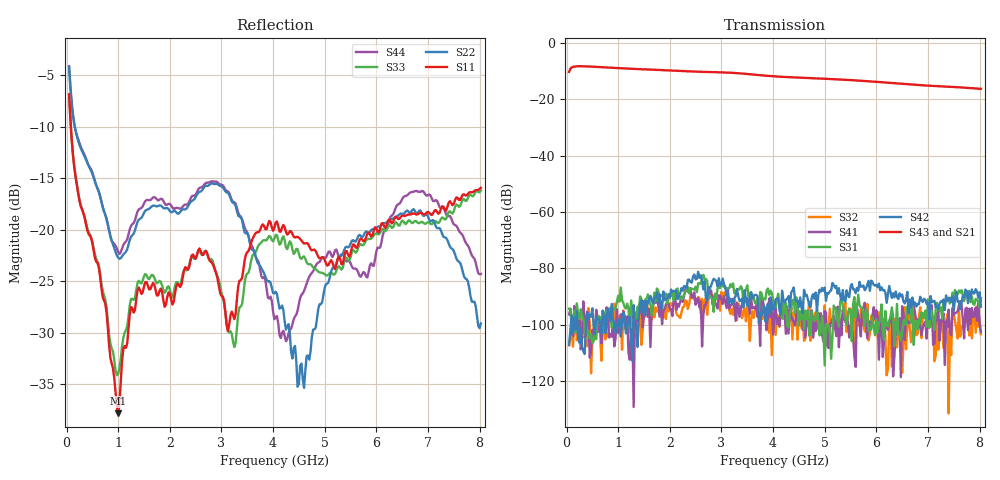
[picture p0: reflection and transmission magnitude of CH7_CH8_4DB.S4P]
!Agilent Technologies,E5071C,MY46316741,A.11.02
!Date: Mon Jun 01 10:29:19 2026
!Data & Calibration Information:
!1:CH7 INPUT 2:CH7 OUTPUT 3:CH8 INPUT 4:CH8 OUTPUT
!Freq	S11:SOLT4(ON)	S12:SOLT4(ON)	S13:SOLT4(ON)	S14:SOLT4(ON)
!	S21:SOLT4(ON)	S22:SOLT4(ON)	S23:SOLT4(ON)	S24:SOLT4(ON)
!	S31:SOLT4(ON)	S32:SOLT4(ON)	S33:SOLT4(ON)	S34:SOLT4(ON)
!	S41:SOLT4(ON)	S42:SOLT4(ON)	S43:SOLT4(ON)	S44:SOLT4(ON)
!PortZ  Port1:50+j0  Port2:50+j0  Port3:50+j0  Port4:50+j0
!Above PortZ is port z conversion or system Z0 setting when saving the data.
!When reading, reference impedance value at option line is always used.
# Hz S dB R 50
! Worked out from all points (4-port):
!   320 points, 50 MHz to 8.025 GHz, reference 50 ohm
!   strongest paths, dB at 50 MHz, 2.05 GHz, 4.05 GHz, 6.05 GHz, 8.025 GHz:
!     S43: -10.2, -9.7, -11.8, -13.8, -16.2
!     S21: -10.3, -9.8, -12.0, -14.0, -16.4
!     S42: -107.1, -88.4, -91.0, -85.4, -93.6
!     S31: -94.4, -88.9, -93.8, -99.3, -90.6
!     S41: -96.4, -97.0, -93.4, -112.5, -102.5
!     S32: -107.4, -93.3, -103.7, -95.6, -103.4
!   lowest |S11| = -37.8 dB at 1 GHz (marker M1), VSWR 1.03, Z = 49.2 - j1 ohm
!   |S11| at or under -10 dB: 84.42 MHz to end of sweep
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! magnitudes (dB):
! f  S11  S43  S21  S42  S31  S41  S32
! 50 MHz  -6.8  -10.2  -10.3  -107.1  -94.4  -96.4  -107.4
! 1 GHz  -37.8  -8.9  -8.9  -100.6  -89.8  -103.0  -98.9
! 1.525 GHz  -25.1  -9.3  -9.4  -96.6  -91.1  -93.1  -97.2
! 3.125 GHz  -29.9  -10.5  -10.6  -88.5  -87.1  -87.6  -90.7
! 4.475 GHz  -20.7  -12.2  -12.4  -91.6  -92.6  -93.5  -105.3
! 6.6 GHz  -18.5  -14.6  -14.8  -88.4  -93.6  -98.6  -100.1
! 8.025 GHz  -15.9  -16.2  -16.4  -93.6  -90.6  -102.5  -103.4
